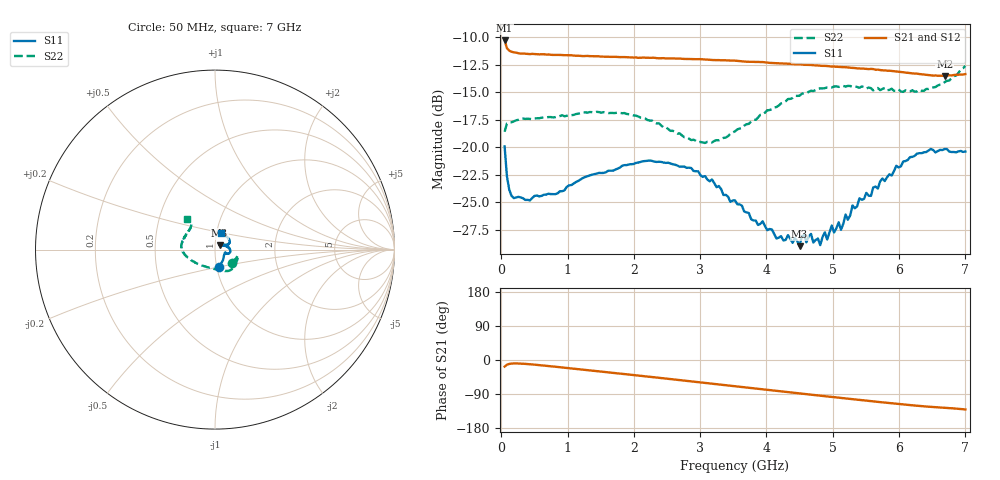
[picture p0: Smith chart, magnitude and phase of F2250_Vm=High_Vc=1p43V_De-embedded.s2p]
! Integrated Device Technology
! Corporate Headquarters
! 6024 Silver Creek Valley Road
! San Jose, CA 95138  USA
! Phone:  1-408-284-8200
! Toll Free:  1-800-223-1366
! Webpage:  http://www.idt.com/
! Timing and RF Division
! 515 Groton Road, Suite 102
! Westford, MA 01886-6024
! Device:  F2250
! Description: Voltage Variable RF Attenuator
! Frequency:  50.0 -  6000.00 MHz
! Package:  3x3 mm Thin QFN Plastic Package: 16 pin
! Ports:  2 RF, 3 DC
!  Pin  1  = GND
!  Pin  2  = NC
!  Pin  3  = RF1  = Port 1
!  Pin  4  = NC
!  Pin  5  = GND
!  Pin  6  = GND
!  Pin  7  = GND
!  Pin  8  = GND
!  Pin  9  = NC
!  Pin 10  = RF2  = Port 2
!  Pin 11  = NC
!  Pin 12  = GND
!  Pin 13  = GND
!  Pin 14  = VCNTRL
!  Pin 15  = VDD
!  Pin 16  = VMODE
! Vcntrl:  1.430 Volts
! Vmode:  +3.300 Volts
! Vdd:  +3.30  Volts
! Current:  1.329 mA
! Data:  The device was measured on a the F2250 evaluation board which has
!  individual transmission lines to the RF pins.  Data was collected
!  using a calibrated network analyzer.  The evaluation board was
!  de-embedded using a TRL calibration technique.
!  The reference plane is the edge of the package pin.
! Misc:  SN 10
!  Action Tracker AT0258
! Date Measured:  2014-11-26
! Date:  2015-10-15  MJV
! Note:
!  Integrated Device Technology supplies this data as a sample of measured
!  data at the package pin for this product.  Your particular data for this
!  product may vary.
!  Data was taken at 25 degrees C.
!  Integrated Device Technology reserves the right to change this data at anytime.
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# GHz S dB R 50
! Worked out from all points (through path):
!   201 points, 50 MHz to 7 GHz, reference 50 ohm
!   highest |S21| = -10.29 dB at 50 MHz (marker M1); lowest = -13.5 dB at 6.687 GHz (marker M2)
!   group delay of S21, straight-line fit = 51.7 ps
!   lowest |S11| = -29.0 dB at 4.498 GHz (marker M3), VSWR 1.07, Z = 52.5 + j2.63 ohm
!   |S11| at or under -10 dB: start of sweep to end of sweep
!   |S22| runs from -19.6 to -12.6 dB; largest |S21 - S12| = 0.0012
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0.05  -19.92 -76.8  -10.29 -17.4  -10.28 -17.3  -18.59 -38.0
0.08475  -22.62 -53.2  -10.99 -12.4  -10.98 -12.4  -17.83 -21.1
0.1195  -23.84 -42.2  -11.22 -10.4  -11.21 -10.4  -17.75 -16.0
0.189  -24.61 -29.1  -11.37 -9.1  -11.38 -9.1  -17.63 -14.2
0.8145  -24.25 -16.5  -11.61 -17.8  -11.61 -17.8  -17.26 -29.8
1.2315  -22.78 -18.5  -11.71 -25.5  -11.70 -25.5  -16.83 -41.6
2.37825  -21.30 -4.4  -11.91 -47.0  -11.92 -47.0  -17.82 -68.2
2.969  -22.18 9.0  -11.99 -58.5  -11.99 -58.5  -19.54 -96.5
3.525  -24.81 24.0  -12.13 -69.3  -12.15 -69.3  -18.55 -133.1
4.1505  -28.28 45.1  -12.36 -81.4  -12.35 -81.4  -16.34 -161.4
4.32425  -27.97 44.2  -12.40 -84.7  -12.40 -84.8  -15.61 -167.0
4.498  -28.97 44.6  -12.45 -88.1  -12.47 -88.1  -15.32 -172.1
4.5675  -27.96 47.8  -12.50 -89.5  -12.50 -89.5  -15.09 -173.2
4.7065  -28.64 48.0  -12.54 -92.1  -12.54 -92.1  -14.89 -176.5
4.81075  -28.88 42.7  -12.59 -94.1  -12.58 -94.1  -14.64 -178.6
5.08875  -26.80 35.2  -12.69 -99.4  -12.69 -99.5  -14.51 174.7
5.1235  -27.48 34.7  -12.71 -100.1  -12.70 -100.2  -14.45 173.8
5.29725  -25.27 26.4  -12.79 -103.3  -12.77 -103.4  -14.52 170.3
5.85325  -22.45 21.3  -13.04 -113.6  -13.04 -113.8  -14.78 155.2
6.27025  -20.57 27.6  -13.31 -120.7  -13.30 -120.8  -14.92 142.2
6.68725  -20.15 44.6  -13.51 -126.1  -13.49 -126.3  -14.08 132.1
7  -20.38 70.7  -13.35 -130.4  -13.35 -130.6  -12.61 132.6
